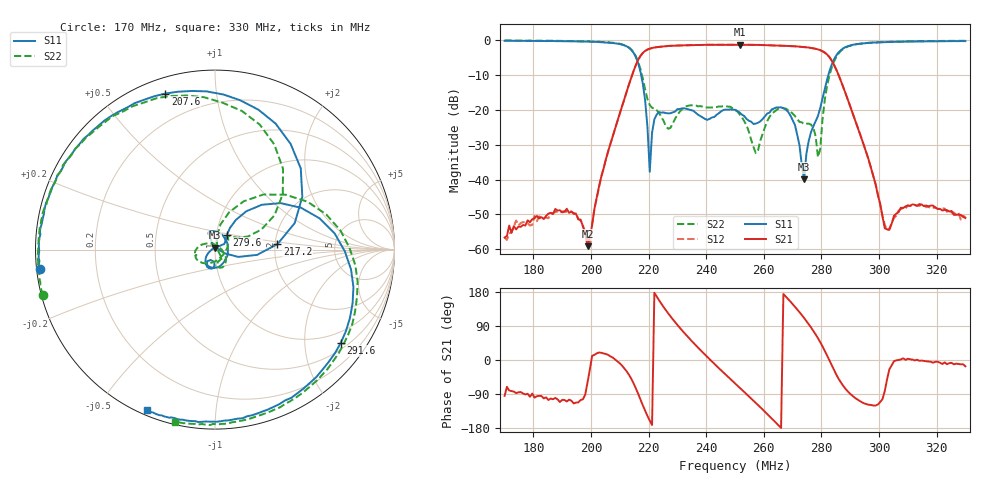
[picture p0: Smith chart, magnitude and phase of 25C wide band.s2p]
!Agilent Technologies,E8362C,SG49020144,A.09.33.09
!Agilent E8362C: A.09.33.09
!Date: Friday, October 10, 2025 10:19:04
!Correction: S11(Full 2 Port(1,2))
!S21(Full 2 Port(1,2))
!S12(Full 2 Port(1,2))
!S22(Full 2 Port(1,2))
!S2P File: Measurements: S11, S21, S12, S22:
# Hz S  dB  R 50
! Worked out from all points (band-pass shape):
!   201 points, 170 MHz to 330 MHz, reference 50 ohm
!   highest |S21| = -1.28 dB at 251.6 MHz (marker M1); lowest = -59.2 dB at 198.8 MHz (marker M2)
!   |S21| within 3 dB of the highest: 217.4 MHz to 282.2 MHz (64.82 MHz wide, 25.9 % of centre)
!   lowest |S11| = -39.9 dB at 274 MHz (marker M3), VSWR 1.02, Z = 50.1 + j1 ohm
!   |S11| at or under -10 dB: 217.4 MHz to 282.4 MHz (65 MHz wide, 26 % of centre)
!   |S22| runs from -33.6 to -0.1 dB; largest |S21 - S12| = 0.0068
!   S11 on the Smith chart (normalised r, x): 170 MHz: 0.01, -0.05; 207.6 MHz: 0.07, +0.73; 217.2 MHz: 2.06, +0.14; 279.6 MHz: 1.13, +0.19; 291.6 MHz: 0.67, -2.89; 330 MHz: 0.02, -0.66
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1.7e8  -0.15 -173.8  -56.66 -94.6  -56.60 -75.9  -0.06 -165.1
1.972e8  -0.36 144.0  -53.47 -103.6  -53.35 -100.1  -0.28 155.0
1.988e8  -0.38 139.9  -59.15 -59.0  -57.34 -60.7  -0.27 151.0
2.076e8  -0.80 107.6  -27.46 6.1  -27.43 5.7  -0.71 119.9
2.172e8  -9.13 5.0  -4.45 -104.8  -4.47 -104.9  -8.35 30.0
2.204e8  -37.79 69.9  -2.40 -160.0  -2.41 -160.2  -18.63 37.6
2.212e8  -26.52 113.6  -2.25 -171.6  -2.21 -171.6  -19.39 45.0
2.236e8  -20.66 106.1  -1.90 157.9  -1.90 158.0  -20.79 35.4
2.3e8  -19.80 110.4  -1.52 92.6  -1.49 92.6  -21.41 -116.0
2.388e8  -22.20 27.6  -1.34 20.0  -1.30 20.0  -19.13 -163.5
2.5e8  -19.97 -111.0  -1.29 -61.8  -1.33 -61.6  -19.96 174.9
2.516e8  -20.76 -119.3  -1.28 -73.0  -1.29 -73.0  -21.31 165.7
2.572e8  -23.94 -107.5  -1.34 -113.1  -1.35 -113.1  -32.40 66.2
2.644e8  -19.31 -100.6  -1.53 -166.9  -1.51 -166.9  -20.06 -58.6
2.708e8  -24.28 -142.3  -1.73 140.8  -1.75 140.5  -21.73 -81.2
2.74e8  -39.92 82.4  -1.97 110.9  -1.97 110.9  -24.11 -59.4
2.772e8  -24.71 30.6  -2.30 76.9  -2.33 76.9  -25.17 -49.6
2.796e8  -19.43 51.2  -2.83 47.0  -2.88 46.9  -31.25 65.9
2.836e8  -6.98 35.3  -5.84 -14.5  -5.88 -14.3  -7.78 48.7
2.916e8  -1.19 -36.6  -22.65 -99.6  -22.71 -99.5  -1.21 -28.4
3.036e8  -0.48 -77.4  -54.46 -24.6  -54.11 -27.1  -0.44 -69.3
3.3e8  -0.25 -112.9  -51.07 -16.6  -50.83 -11.8  -0.14 -103.1
